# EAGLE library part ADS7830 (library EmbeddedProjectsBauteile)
Texas Instruments 8-Bit, 8-Channel Sampling ANALOG-TO-DIGITAL CONVERTER with I2CTM Interface
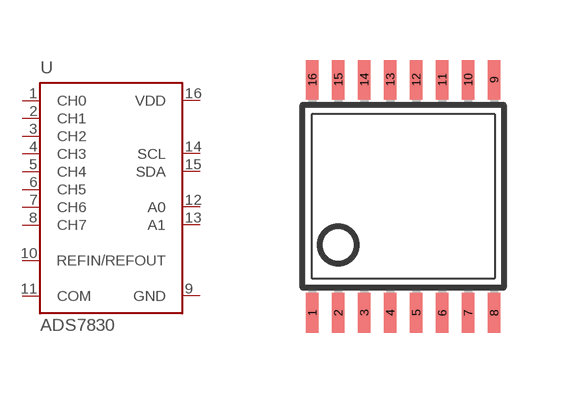
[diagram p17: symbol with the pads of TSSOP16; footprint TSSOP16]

Designator prefix -

## ADS7830 (EP: 400855)  [TSSOP16]
1  CH0  in
2  CH1  in
3  CH2  in
4  CH3  in
5  CH4  in
6  CH5  in
7  CH6  in
8  CH7  in
9  GND  pwr
10  REFIN/REFOUT  pas
11  COM  in
12  A0  in
13  A1  in
14  SCL  in
15  SDA
16  VDD  pwr

## Footprint TSSOP16 (pad centres in mm)
smd 0.305 x 0.991: 1 -2.275,-2.918; 2 -1.625,-2.918; 3 -0.975,-2.918; 4 -0.325,-2.918; 5 0.325,-2.918; 6 0.975,-2.918; 7 1.625,-2.918; 8 2.275,-2.918; 9 2.275,2.918; 10 1.625,2.918; 11 0.975,2.918; 12 0.325,2.918; 13 -0.325,2.918; 14 -0.975,2.918; 15 -1.625,2.918; 16 -2.275,2.918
